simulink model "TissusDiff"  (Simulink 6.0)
settings: Solver=ode45  StartTime=0.0  StopTime=15  RelTol=1e-3
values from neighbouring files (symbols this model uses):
  b = S/Sm    (= 0.1)    [Constantes.m]    (also in ConstantesBck.m)
  C = 1    [Constantes.m]    (also in ConstantesBck.m)
  gk = 36    [Constantes.m]    (also in ConstantesBck.m; sim_hh.m)
  gl = 0.3    [Constantes.m]    (also in ConstantesBck.m; sim_hh.m)
  gna = 120    [Constantes.m]    (also in ConstantesBck.m; sim_hh.m)
  h0 = 0.5961    [Constantes.m]    (also in ConstantesBck.m)
  Istim = 200E-6    (= 0.0002)    [Constantes.m]    (also in ConstantesBck.m = 5e-05)
  m0 = 0.0529    [Constantes.m]    (also in ConstantesBck.m)
  mK = 0    [Constantes.m]    (also in ConstantesBck.m)
  mL = 0    [Constantes.m]    (also in ConstantesBck.m)
  mNa = 0    [Constantes.m]    (also in ConstantesBck.m)
  n0 = 0.3177    [Constantes.m]    (also in ConstantesBck.m)
  rapportIE = 10    [Constantes.m]
  Rext = 2.9E3    (= 2900)    [Constantes.m]    (also in ConstantesBck.m)
  Rint = 2.9E2    (= 290)    [Constantes.m]    (also in ConstantesBck.m = 400)
  Sm = 3.14e-2    (= 0.0314)    [Constantes.m]    (also in ConstantesBck.m = 0.000314)
  Vk = -82    [Constantes.m]    (also in ConstantesBck.m)
  Vl = -59    [Constantes.m]    (also in ConstantesBck.m)
  Vna = 45    [Constantes.m]    (also in ConstantesBck.m)
  Vr = -70    [Constantes.m]    (also in ConstantesBck.m)
undefined symbols (not defined in the file or in its folder): ln

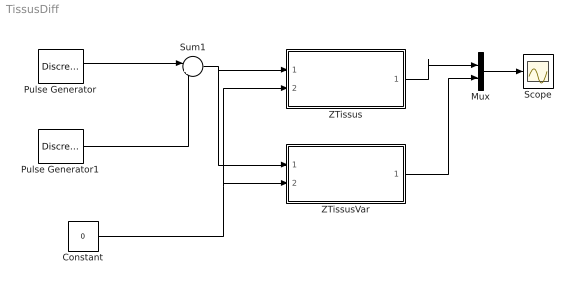
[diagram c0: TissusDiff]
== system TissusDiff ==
  Constant : Constant  Value=0
  Mux : Mux  Inputs=2
  Pulse Generator : DiscretePulseGenerator  PulseType=Time based  Amplitude=-Istim  Period=100  PulseWidth=2  PhaseDelay=2
  Pulse Generator1 : DiscretePulseGenerator  PulseType=Time based  Amplitude=Istim  Period=100  PulseWidth=2  PhaseDelay=4
  Scope : Scope
  Sum1 : Sum  Inputs=|++
  ZTissus : Subsystem
  ZTissusVar : Subsystem
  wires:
  Pulse Generator/1 -> Sum1/1
  Pulse Generator1/1 -> Sum1/2
  Constant/1 -> ZTissus/2(Vref), ZTissusVar/2(Vref)
  Mux/1 -> Scope/1
  Sum1/1 -> ZTissusVar/1(IStim), ZTissus/1(IStim)
  ZTissusVar/1(Vout) -> Mux/2
  ZTissus/1(Vout) -> Mux/1

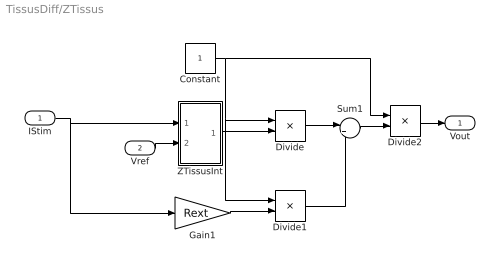
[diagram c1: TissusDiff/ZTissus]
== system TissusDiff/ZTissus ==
  IStim : Inport  Port=1  LatchInput=off
  Vref : Inport  Port=2  LatchInput=off
  Constant : Constant
  Divide : Product  Inputs=*/  OutScaling=2^-10
  Divide1 : Product  Inputs=*/  OutScaling=2^-10
  Divide2 : Product  Inputs=*/  OutScaling=2^-10
  Gain1 : Gain  Gain=Rext
  Sum1 : Sum  Inputs=|++
  ZTissusInt : Subsystem
  Vout : Outport
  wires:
  IStim/1 -> ZTissusInt/1(InStim), Gain1/1
  Constant/1 -> Divide/1, Divide1/1, Divide2/1
  ZTissusInt/1(Vout) -> Divide/2
  Gain1/1 -> Divide1/2
  Divide/1 -> Sum1/1
  Divide1/1 -> Sum1/2
  Sum1/1 -> Divide2/2
  Divide2/1 -> Vout/1
  Vref/1 -> ZTissusInt/2(VRefIn)

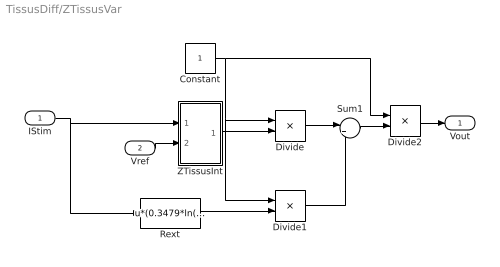
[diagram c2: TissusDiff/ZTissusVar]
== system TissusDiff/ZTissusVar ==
  IStim : Inport  Port=1  LatchInput=off
  Vref : Inport  Port=2  LatchInput=off
  Constant : Constant
  Divide : Product  Inputs=*/  OutScaling=2^-10
  Divide1 : Product  Inputs=*/  OutScaling=2^-10
  Divide2 : Product  Inputs=*/  OutScaling=2^-10
  Rext : Fcn  Expr=u*(0.3479*ln(abs(u)*1E6)+1.3815)*1E3
  Sum1 : Sum  Inputs=|++
  ZTissusInt : Subsystem
  Vout : Outport
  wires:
  IStim/1 -> ZTissusInt/1(InStim), Rext/1
  Constant/1 -> Divide/1, Divide1/1, Divide2/1
  ZTissusInt/1(Vout) -> Divide/2
  Rext/1 -> Divide1/2
  Divide/1 -> Sum1/1
  Divide1/1 -> Sum1/2
  Sum1/1 -> Divide2/2
  Divide2/1 -> Vout/1
  Vref/1 -> ZTissusInt/2(VRefIn)

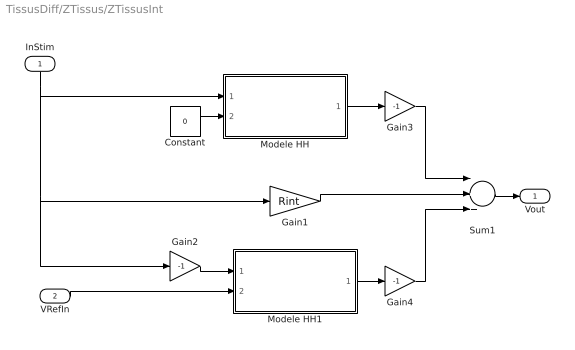
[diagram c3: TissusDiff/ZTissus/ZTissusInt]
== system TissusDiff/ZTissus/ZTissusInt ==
  InStim : Inport  Orientation=down  Port=1  LatchInput=off
  VRefIn : Inport  Port=2  LatchInput=off
  Constant : Constant  Value=0
  Gain1 : Gain  Gain=Rint
  Gain2 : Gain  Gain=-1
  Gain3 : Gain  Gain=-1
  Gain4 : Gain  Gain=-1
  Modele HH : Subsystem
  Modele HH1 : Subsystem
  Sum1 : Sum  Inputs=|+++
  Vout : Outport
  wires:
  Modele HH/1(HHout) -> Gain3/1
  Modele HH1/1(HHout) -> Gain4/1
  Gain1/1 -> Sum1/2
  Gain2/1 -> Modele HH1/1(HHin)
  InStim/1 -> Gain1/1, Gain2/1, Modele HH/1(HHin)
  Constant/1 -> Modele HH/2(VRefIn)
  Sum1/1 -> Vout/1
  VRefIn/1 -> Modele HH1/2(VRefIn)
  Gain3/1 -> Sum1/1
  Gain4/1 -> Sum1/3

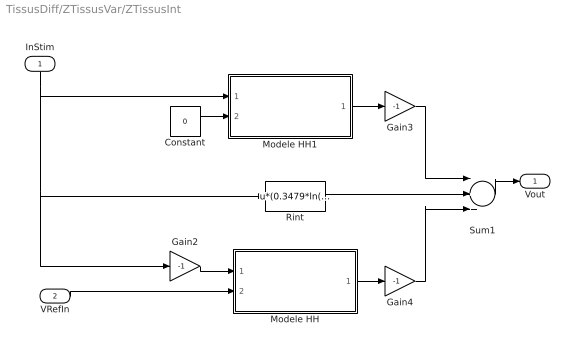
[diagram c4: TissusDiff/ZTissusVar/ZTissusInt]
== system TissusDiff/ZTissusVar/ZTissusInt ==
  InStim : Inport  Orientation=down  Port=1  LatchInput=off
  VRefIn : Inport  Port=2  LatchInput=off
  Constant : Constant  Value=0
  Gain2 : Gain  Gain=-1
  Gain3 : Gain  Gain=-1
  Gain4 : Gain  Gain=-1
  Modele HH : Subsystem
  Modele HH1 : Subsystem
  Rint : Fcn  Expr=u*(0.3479*ln(abs(u)*1E6)+1.3815)*1E3/rapportIE
  Sum1 : Sum  Inputs=|+++
  Vout : Outport
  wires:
  Modele HH1/1(HHout) -> Gain3/1
  Modele HH/1(HHout) -> Gain4/1
  Rint/1 -> Sum1/2
  Gain2/1 -> Modele HH/1(HHin)
  InStim/1 -> Gain2/1, Rint/1, Modele HH1/1(HHin)
  Constant/1 -> Modele HH1/2(VRefIn)
  Sum1/1 -> Vout/1
  VRefIn/1 -> Modele HH/2(VRefIn)
  Gain3/1 -> Sum1/1
  Gain4/1 -> Sum1/3

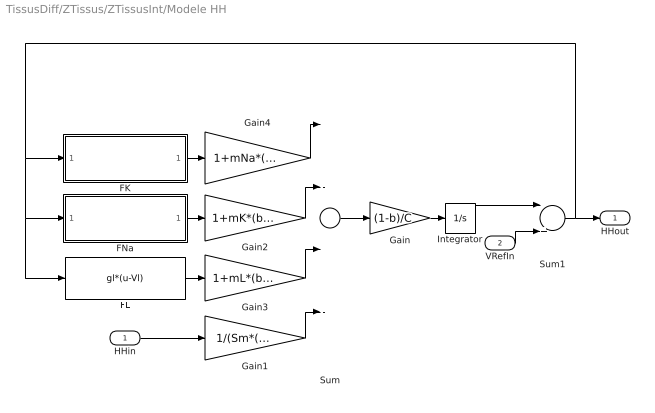
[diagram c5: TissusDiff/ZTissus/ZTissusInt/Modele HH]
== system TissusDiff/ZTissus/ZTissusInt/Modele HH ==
  HHin : Inport  Port=1  LatchInput=off
  VRefIn : Inport  Port=2  LatchInput=off
  FK : Subsystem
  FL : Fcn  Expr=gl*(u-Vl)
  FNa : Subsystem
  Gain : Gain  Gain=(1-b)/C
  Gain1 : Gain  Gain=1/(Sm*(1-b))
  Gain2 : Gain  Gain=1+mK*(b/(1-b))
  Gain3 : Gain  Gain=1+mL*(b/(1-b))
  Gain4 : Gain  Gain=1+mNa*(b/(1-b))
  Integrator : Integrator  InitialCondition=Vr
  Sum : Sum  Inputs=|---+
  Sum1 : Sum  Inputs=|++
  HHout : Outport
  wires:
  Sum/1 -> Gain/1
  Gain/1 -> Integrator/1
  FK/1(FKout) -> Gain4/1
  FNa/1(FNaOut) -> Gain2/1
  FL/1 -> Gain3/1
  HHin/1 -> Gain1/1
  Integrator/1 -> Sum1/1
  Sum1/1 -> HHout/1, FNa/1(FNaIn), FL/1, FK/1(FKIn)
  VRefIn/1 -> Sum1/2
  Gain1/1 -> Sum/4
  Gain4/1 -> Sum/1
  Gain2/1 -> Sum/2
  Gain3/1 -> Sum/3

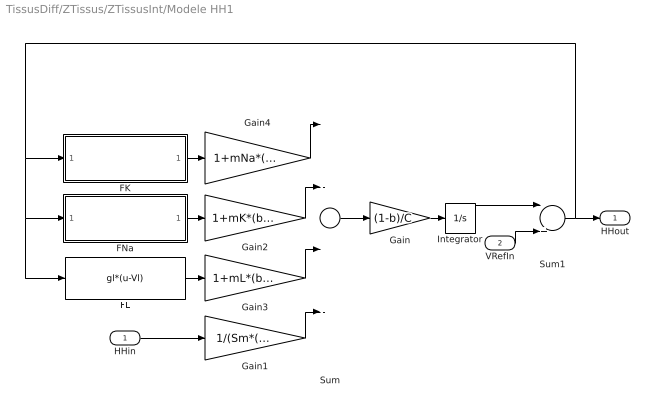
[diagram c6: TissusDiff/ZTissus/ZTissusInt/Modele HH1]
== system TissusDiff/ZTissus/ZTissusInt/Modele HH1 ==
  HHin : Inport  Port=1  LatchInput=off
  VRefIn : Inport  Port=2  LatchInput=off
  FK : Subsystem
  FL : Fcn  Expr=gl*(u-Vl)
  FNa : Subsystem
  Gain : Gain  Gain=(1-b)/C
  Gain1 : Gain  Gain=1/(Sm*(1-b))
  Gain2 : Gain  Gain=1+mK*(b/(1-b))
  Gain3 : Gain  Gain=1+mL*(b/(1-b))
  Gain4 : Gain  Gain=1+mNa*(b/(1-b))
  Integrator : Integrator  InitialCondition=Vr
  Sum : Sum  Inputs=|---+
  Sum1 : Sum  Inputs=|++
  HHout : Outport
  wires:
  Sum/1 -> Gain/1
  Gain/1 -> Integrator/1
  FK/1(FKout) -> Gain4/1
  FNa/1(FNaOut) -> Gain2/1
  FL/1 -> Gain3/1
  HHin/1 -> Gain1/1
  Integrator/1 -> Sum1/1
  Sum1/1 -> HHout/1, FNa/1(FNaIn), FL/1, FK/1(FKIn)
  VRefIn/1 -> Sum1/2
  Gain1/1 -> Sum/4
  Gain4/1 -> Sum/1
  Gain2/1 -> Sum/2
  Gain3/1 -> Sum/3

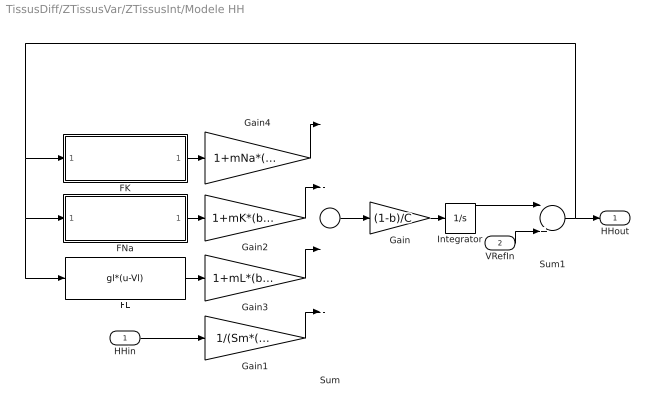
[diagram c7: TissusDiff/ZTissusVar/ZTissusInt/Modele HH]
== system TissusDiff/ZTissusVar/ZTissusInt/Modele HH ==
  HHin : Inport  Port=1  LatchInput=off
  VRefIn : Inport  Port=2  LatchInput=off
  FK : Subsystem
  FL : Fcn  Expr=gl*(u-Vl)
  FNa : Subsystem
  Gain : Gain  Gain=(1-b)/C
  Gain1 : Gain  Gain=1/(Sm*(1-b))
  Gain2 : Gain  Gain=1+mK*(b/(1-b))
  Gain3 : Gain  Gain=1+mL*(b/(1-b))
  Gain4 : Gain  Gain=1+mNa*(b/(1-b))
  Integrator : Integrator  InitialCondition=Vr
  Sum : Sum  Inputs=|---+
  Sum1 : Sum  Inputs=|++
  HHout : Outport
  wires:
  Sum/1 -> Gain/1
  Gain/1 -> Integrator/1
  FK/1(FKout) -> Gain4/1
  FNa/1(FNaOut) -> Gain2/1
  FL/1 -> Gain3/1
  HHin/1 -> Gain1/1
  Integrator/1 -> Sum1/1
  Sum1/1 -> HHout/1, FNa/1(FNaIn), FL/1, FK/1(FKIn)
  VRefIn/1 -> Sum1/2
  Gain1/1 -> Sum/4
  Gain4/1 -> Sum/1
  Gain2/1 -> Sum/2
  Gain3/1 -> Sum/3

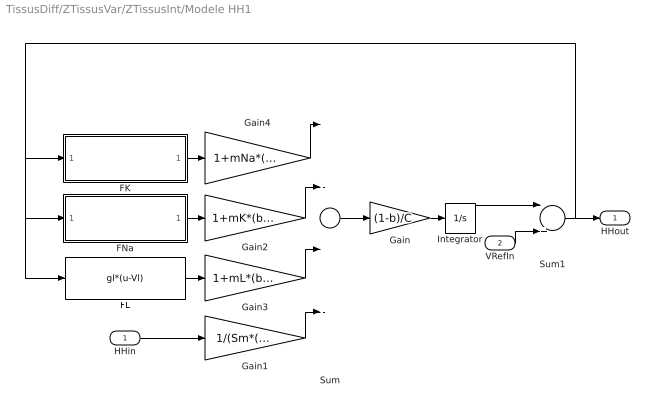
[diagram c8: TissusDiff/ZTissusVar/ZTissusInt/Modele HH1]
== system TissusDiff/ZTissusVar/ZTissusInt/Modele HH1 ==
  HHin : Inport  Port=1  LatchInput=off
  VRefIn : Inport  Port=2  LatchInput=off
  FK : Subsystem
  FL : Fcn  Expr=gl*(u-Vl)
  FNa : Subsystem
  Gain : Gain  Gain=(1-b)/C
  Gain1 : Gain  Gain=1/(Sm*(1-b))
  Gain2 : Gain  Gain=1+mK*(b/(1-b))
  Gain3 : Gain  Gain=1+mL*(b/(1-b))
  Gain4 : Gain  Gain=1+mNa*(b/(1-b))
  Integrator : Integrator  InitialCondition=Vr
  Sum : Sum  Inputs=|---+
  Sum1 : Sum  Inputs=|++
  HHout : Outport
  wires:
  Sum/1 -> Gain/1
  Gain/1 -> Integrator/1
  FK/1(FKout) -> Gain4/1
  FNa/1(FNaOut) -> Gain2/1
  FL/1 -> Gain3/1
  HHin/1 -> Gain1/1
  Integrator/1 -> Sum1/1
  Sum1/1 -> HHout/1, FNa/1(FNaIn), FL/1, FK/1(FKIn)
  VRefIn/1 -> Sum1/2
  Gain1/1 -> Sum/4
  Gain4/1 -> Sum/1
  Gain2/1 -> Sum/2
  Gain3/1 -> Sum/3

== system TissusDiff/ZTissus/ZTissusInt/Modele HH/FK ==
  note: gkm
  note: (Vm-Vk0)
  FKIn : Inport  Port=1  LatchInput=off
  (Vm-Vk0) : Fcn  Expr=(u-Vk)
  Product : Product
  n(Vm) : Subsystem
  n^4 : Fcn  Expr=gk*(u^4)
  FKout : Outport  InitialOutput=0
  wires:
  n(Vm)/1(n) -> n^4/1
  (Vm-Vk0)/1 -> Product/2
  Product/1 -> FKout/1
  n^4/1 -> Product/1
  FKIn/1 -> n(Vm)/1(Vm), (Vm-Vk0)/1

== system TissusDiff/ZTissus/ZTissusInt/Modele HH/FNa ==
  note: gNa*m^3
  note: m
  note: h
  note: gNam
  note: (Vm-VNa0)
  FNaIn : Inport  Port=1  LatchInput=off
  (Vm-VNa0) : Fcn  Expr=(u-Vna)
  Product : Product
  Product1 : Product
  gna*m^3 : Fcn  Expr=gna*u^3
  h(Vm) : Subsystem
  m(Vm) : Subsystem
  FNaOut : Outport  InitialOutput=0
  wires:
  (Vm-VNa0)/1 -> Product1/2
  gna*m^3/1 -> Product/1
  Product1/1 -> FNaOut/1
  FNaIn/1 -> m(Vm)/1(Vm), h(Vm)/1(Vm), (Vm-VNa0)/1
  m(Vm)/1(n) -> gna*m^3/1
  h(Vm)/1(h) -> Product/2
  Product/1 -> Product1/1

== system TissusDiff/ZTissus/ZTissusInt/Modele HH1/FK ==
  note: gkm
  note: (Vm-Vk0)
  FKIn : Inport  Port=1  LatchInput=off
  (Vm-Vk0) : Fcn  Expr=(u-Vk)
  Product : Product
  n(Vm) : Subsystem
  n^4 : Fcn  Expr=gk*(u^4)
  FKout : Outport  InitialOutput=0
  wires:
  n(Vm)/1(n) -> n^4/1
  (Vm-Vk0)/1 -> Product/2
  Product/1 -> FKout/1
  n^4/1 -> Product/1
  FKIn/1 -> n(Vm)/1(Vm), (Vm-Vk0)/1

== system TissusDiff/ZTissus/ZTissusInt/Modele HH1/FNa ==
  note: gNa*m^3
  note: m
  note: h
  note: gNam
  note: (Vm-VNa0)
  FNaIn : Inport  Port=1  LatchInput=off
  (Vm-VNa0) : Fcn  Expr=(u-Vna)
  Product : Product
  Product1 : Product
  gna*m^3 : Fcn  Expr=gna*u^3
  h(Vm) : Subsystem
  m(Vm) : Subsystem
  FNaOut : Outport  InitialOutput=0
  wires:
  (Vm-VNa0)/1 -> Product1/2
  gna*m^3/1 -> Product/1
  Product1/1 -> FNaOut/1
  FNaIn/1 -> m(Vm)/1(Vm), h(Vm)/1(Vm), (Vm-VNa0)/1
  m(Vm)/1(n) -> gna*m^3/1
  h(Vm)/1(h) -> Product/2
  Product/1 -> Product1/1

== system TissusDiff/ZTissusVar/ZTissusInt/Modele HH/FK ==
  note: gkm
  note: (Vm-Vk0)
  FKIn : Inport  Port=1  LatchInput=off
  (Vm-Vk0) : Fcn  Expr=(u-Vk)
  Product : Product
  n(Vm) : Subsystem
  n^4 : Fcn  Expr=gk*(u^4)
  FKout : Outport  InitialOutput=0
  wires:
  n(Vm)/1(n) -> n^4/1
  (Vm-Vk0)/1 -> Product/2
  Product/1 -> FKout/1
  n^4/1 -> Product/1
  FKIn/1 -> n(Vm)/1(Vm), (Vm-Vk0)/1

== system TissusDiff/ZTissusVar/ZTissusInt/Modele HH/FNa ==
  note: gNa*m^3
  note: m
  note: h
  note: gNam
  note: (Vm-VNa0)
  FNaIn : Inport  Port=1  LatchInput=off
  (Vm-VNa0) : Fcn  Expr=(u-Vna)
  Product : Product
  Product1 : Product
  gna*m^3 : Fcn  Expr=gna*u^3
  h(Vm) : Subsystem
  m(Vm) : Subsystem
  FNaOut : Outport  InitialOutput=0
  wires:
  (Vm-VNa0)/1 -> Product1/2
  gna*m^3/1 -> Product/1
  Product1/1 -> FNaOut/1
  FNaIn/1 -> m(Vm)/1(Vm), h(Vm)/1(Vm), (Vm-VNa0)/1
  m(Vm)/1(n) -> gna*m^3/1
  h(Vm)/1(h) -> Product/2
  Product/1 -> Product1/1

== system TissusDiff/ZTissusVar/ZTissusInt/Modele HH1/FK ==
  note: gkm
  note: (Vm-Vk0)
  FKIn : Inport  Port=1  LatchInput=off
  (Vm-Vk0) : Fcn  Expr=(u-Vk)
  Product : Product
  n(Vm) : Subsystem
  n^4 : Fcn  Expr=gk*(u^4)
  FKout : Outport  InitialOutput=0
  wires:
  n(Vm)/1(n) -> n^4/1
  (Vm-Vk0)/1 -> Product/2
  Product/1 -> FKout/1
  n^4/1 -> Product/1
  FKIn/1 -> n(Vm)/1(Vm), (Vm-Vk0)/1

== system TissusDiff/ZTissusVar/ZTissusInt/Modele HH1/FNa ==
  note: gNa*m^3
  note: m
  note: h
  note: gNam
  note: (Vm-VNa0)
  FNaIn : Inport  Port=1  LatchInput=off
  (Vm-VNa0) : Fcn  Expr=(u-Vna)
  Product : Product
  Product1 : Product
  gna*m^3 : Fcn  Expr=gna*u^3
  h(Vm) : Subsystem
  m(Vm) : Subsystem
  FNaOut : Outport  InitialOutput=0
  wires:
  (Vm-VNa0)/1 -> Product1/2
  gna*m^3/1 -> Product/1
  Product1/1 -> FNaOut/1
  FNaIn/1 -> m(Vm)/1(Vm), h(Vm)/1(Vm), (Vm-VNa0)/1
  m(Vm)/1(n) -> gna*m^3/1
  h(Vm)/1(h) -> Product/2
  Product/1 -> Product1/1

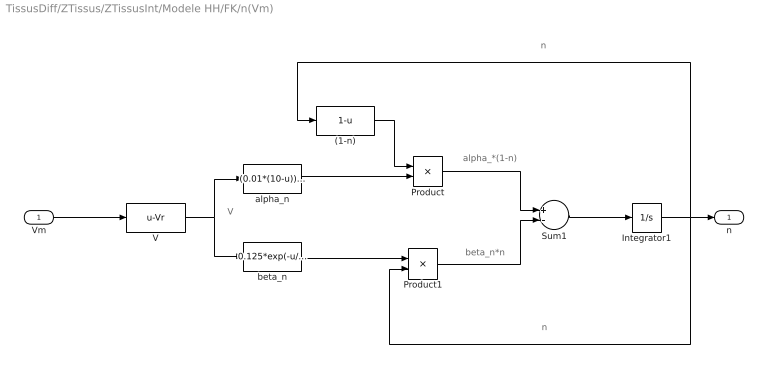
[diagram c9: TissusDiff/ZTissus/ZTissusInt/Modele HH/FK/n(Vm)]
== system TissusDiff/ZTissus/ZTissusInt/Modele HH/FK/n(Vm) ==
  note: V
  note: alpha_*(1-n)
  note: beta_n*n
  note: n
  note: n
  Vm : Inport  Port=1  LatchInput=off
  (1-n) : Fcn  Expr=1-u
  Integrator1 : Integrator  InitialCondition=n0
  Product : Product
  Product1 : Product
  Sum1 : Sum  Inputs=+-
  V : Fcn  Expr=u-Vr
  alpha_n : Fcn  Expr=(0.01*(10-u))/(exp((10-u)/10)-1)
  beta_n : Fcn  Expr=0.125*exp(-u/80)
  n : Outport  InitialOutput=0
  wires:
  V/1 -> alpha_n/1, beta_n/1
  alpha_n/1 -> Product/2
  (1-n)/1 -> Product/1
  beta_n/1 -> Product1/1
  Product/1 -> Sum1/1
  Product1/1 -> Sum1/2
  Sum1/1 -> Integrator1/1
  Integrator1/1 -> (1-n)/1, Product1/2, n/1
  Vm/1 -> V/1

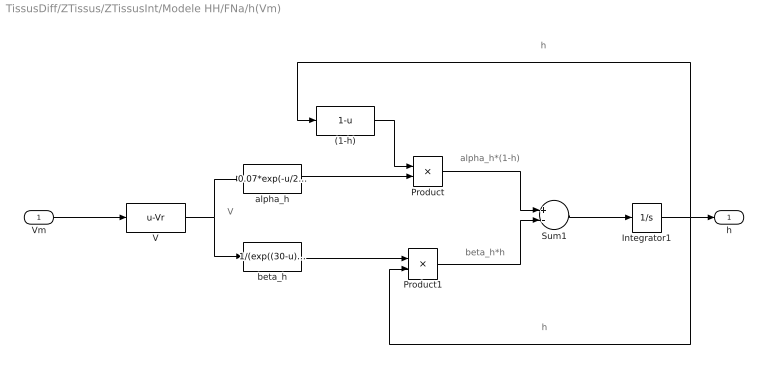
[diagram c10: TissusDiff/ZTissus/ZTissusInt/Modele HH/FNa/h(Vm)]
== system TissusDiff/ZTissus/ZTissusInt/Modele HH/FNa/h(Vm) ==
  note: h
  note: h
  note: beta_h*h
  note: alpha_h*(1-h)
  note: V
  Vm : Inport  Port=1  LatchInput=off
  (1-h) : Fcn  Expr=1-u
  Integrator1 : Integrator  InitialCondition=h0
  Product : Product
  Product1 : Product
  Sum1 : Sum  Inputs=+-
  V : Fcn  Expr=u-Vr
  alpha_h : Fcn  Expr=0.07*exp(-u/20)
  beta_h : Fcn  Expr=1/(exp((30-u)/10)+1)
  h : Outport  InitialOutput=0
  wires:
  Vm/1 -> V/1
  Integrator1/1 -> h/1, Product1/2, (1-h)/1
  Sum1/1 -> Integrator1/1
  Product1/1 -> Sum1/2
  Product/1 -> Sum1/1
  beta_h/1 -> Product1/1
  (1-h)/1 -> Product/1
  alpha_h/1 -> Product/2
  V/1 -> beta_h/1, alpha_h/1

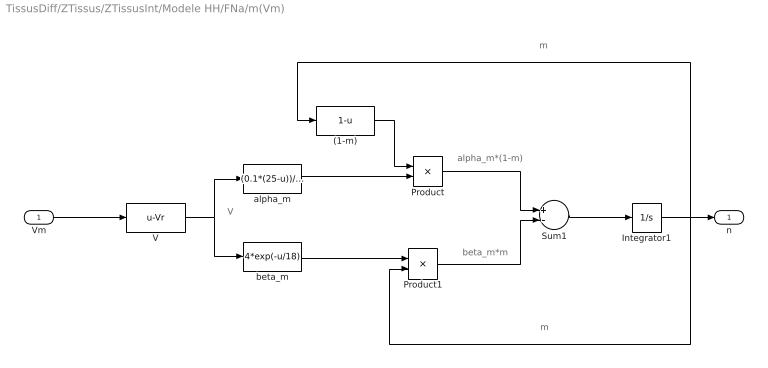
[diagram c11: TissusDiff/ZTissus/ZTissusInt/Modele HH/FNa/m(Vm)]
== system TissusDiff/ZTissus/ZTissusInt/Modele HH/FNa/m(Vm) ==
  note: m
  note: m
  note: beta_m*m
  note: alpha_m*(1-m)
  note: V
  Vm : Inport  Port=1  LatchInput=off
  (1-m) : Fcn  Expr=1-u
  Integrator1 : Integrator  InitialCondition=m0
  Product : Product
  Product1 : Product
  Sum1 : Sum  Inputs=+-
  V : Fcn  Expr=u-Vr
  alpha_m : Fcn  Expr=(0.1*(25-u))/(exp((25-u)/10)-1)
  beta_m : Fcn  Expr=4*exp(-u/18)
  n : Outport  InitialOutput=0
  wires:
  Vm/1 -> V/1
  Integrator1/1 -> n/1, Product1/2, (1-m)/1
  Sum1/1 -> Integrator1/1
  Product1/1 -> Sum1/2
  Product/1 -> Sum1/1
  beta_m/1 -> Product1/1
  (1-m)/1 -> Product/1
  alpha_m/1 -> Product/2
  V/1 -> beta_m/1, alpha_m/1

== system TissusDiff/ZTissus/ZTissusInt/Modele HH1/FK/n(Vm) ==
  note: V
  note: alpha_*(1-n)
  note: beta_n*n
  note: n
  note: n
  Vm : Inport  Port=1  LatchInput=off
  (1-n) : Fcn  Expr=1-u
  Integrator1 : Integrator  InitialCondition=n0
  Product : Product
  Product1 : Product
  Sum1 : Sum  Inputs=+-
  V : Fcn  Expr=u-Vr
  alpha_n : Fcn  Expr=(0.01*(10-u))/(exp((10-u)/10)-1)
  beta_n : Fcn  Expr=0.125*exp(-u/80)
  n : Outport  InitialOutput=0
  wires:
  V/1 -> alpha_n/1, beta_n/1
  alpha_n/1 -> Product/2
  (1-n)/1 -> Product/1
  beta_n/1 -> Product1/1
  Product/1 -> Sum1/1
  Product1/1 -> Sum1/2
  Sum1/1 -> Integrator1/1
  Integrator1/1 -> (1-n)/1, Product1/2, n/1
  Vm/1 -> V/1

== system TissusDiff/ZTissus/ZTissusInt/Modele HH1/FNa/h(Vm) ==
  note: h
  note: h
  note: beta_h*h
  note: alpha_h*(1-h)
  note: V
  Vm : Inport  Port=1  LatchInput=off
  (1-h) : Fcn  Expr=1-u
  Integrator1 : Integrator  InitialCondition=h0
  Product : Product
  Product1 : Product
  Sum1 : Sum  Inputs=+-
  V : Fcn  Expr=u-Vr
  alpha_h : Fcn  Expr=0.07*exp(-u/20)
  beta_h : Fcn  Expr=1/(exp((30-u)/10)+1)
  h : Outport  InitialOutput=0
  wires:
  Vm/1 -> V/1
  Integrator1/1 -> h/1, Product1/2, (1-h)/1
  Sum1/1 -> Integrator1/1
  Product1/1 -> Sum1/2
  Product/1 -> Sum1/1
  beta_h/1 -> Product1/1
  (1-h)/1 -> Product/1
  alpha_h/1 -> Product/2
  V/1 -> beta_h/1, alpha_h/1

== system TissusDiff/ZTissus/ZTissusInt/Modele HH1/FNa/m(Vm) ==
  note: m
  note: m
  note: beta_m*m
  note: alpha_m*(1-m)
  note: V
  Vm : Inport  Port=1  LatchInput=off
  (1-m) : Fcn  Expr=1-u
  Integrator1 : Integrator  InitialCondition=m0
  Product : Product
  Product1 : Product
  Sum1 : Sum  Inputs=+-
  V : Fcn  Expr=u-Vr
  alpha_m : Fcn  Expr=(0.1*(25-u))/(exp((25-u)/10)-1)
  beta_m : Fcn  Expr=4*exp(-u/18)
  n : Outport  InitialOutput=0
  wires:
  Vm/1 -> V/1
  Integrator1/1 -> n/1, Product1/2, (1-m)/1
  Sum1/1 -> Integrator1/1
  Product1/1 -> Sum1/2
  Product/1 -> Sum1/1
  beta_m/1 -> Product1/1
  (1-m)/1 -> Product/1
  alpha_m/1 -> Product/2
  V/1 -> beta_m/1, alpha_m/1

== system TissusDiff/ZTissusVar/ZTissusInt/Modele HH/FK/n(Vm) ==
  note: V
  note: alpha_*(1-n)
  note: beta_n*n
  note: n
  note: n
  Vm : Inport  Port=1  LatchInput=off
  (1-n) : Fcn  Expr=1-u
  Integrator1 : Integrator  InitialCondition=n0
  Product : Product
  Product1 : Product
  Sum1 : Sum  Inputs=+-
  V : Fcn  Expr=u-Vr
  alpha_n : Fcn  Expr=(0.01*(10-u))/(exp((10-u)/10)-1)
  beta_n : Fcn  Expr=0.125*exp(-u/80)
  n : Outport  InitialOutput=0
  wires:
  V/1 -> alpha_n/1, beta_n/1
  alpha_n/1 -> Product/2
  (1-n)/1 -> Product/1
  beta_n/1 -> Product1/1
  Product/1 -> Sum1/1
  Product1/1 -> Sum1/2
  Sum1/1 -> Integrator1/1
  Integrator1/1 -> (1-n)/1, Product1/2, n/1
  Vm/1 -> V/1

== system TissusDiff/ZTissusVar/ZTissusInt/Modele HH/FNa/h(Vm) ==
  note: h
  note: h
  note: beta_h*h
  note: alpha_h*(1-h)
  note: V
  Vm : Inport  Port=1  LatchInput=off
  (1-h) : Fcn  Expr=1-u
  Integrator1 : Integrator  InitialCondition=h0
  Product : Product
  Product1 : Product
  Sum1 : Sum  Inputs=+-
  V : Fcn  Expr=u-Vr
  alpha_h : Fcn  Expr=0.07*exp(-u/20)
  beta_h : Fcn  Expr=1/(exp((30-u)/10)+1)
  h : Outport  InitialOutput=0
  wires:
  Vm/1 -> V/1
  Integrator1/1 -> h/1, Product1/2, (1-h)/1
  Sum1/1 -> Integrator1/1
  Product1/1 -> Sum1/2
  Product/1 -> Sum1/1
  beta_h/1 -> Product1/1
  (1-h)/1 -> Product/1
  alpha_h/1 -> Product/2
  V/1 -> beta_h/1, alpha_h/1

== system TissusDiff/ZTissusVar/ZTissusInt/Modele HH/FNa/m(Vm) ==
  note: m
  note: m
  note: beta_m*m
  note: alpha_m*(1-m)
  note: V
  Vm : Inport  Port=1  LatchInput=off
  (1-m) : Fcn  Expr=1-u
  Integrator1 : Integrator  InitialCondition=m0
  Product : Product
  Product1 : Product
  Sum1 : Sum  Inputs=+-
  V : Fcn  Expr=u-Vr
  alpha_m : Fcn  Expr=(0.1*(25-u))/(exp((25-u)/10)-1)
  beta_m : Fcn  Expr=4*exp(-u/18)
  n : Outport  InitialOutput=0
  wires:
  Vm/1 -> V/1
  Integrator1/1 -> n/1, Product1/2, (1-m)/1
  Sum1/1 -> Integrator1/1
  Product1/1 -> Sum1/2
  Product/1 -> Sum1/1
  beta_m/1 -> Product1/1
  (1-m)/1 -> Product/1
  alpha_m/1 -> Product/2
  V/1 -> beta_m/1, alpha_m/1

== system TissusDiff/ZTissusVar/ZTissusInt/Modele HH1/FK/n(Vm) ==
  note: V
  note: alpha_*(1-n)
  note: beta_n*n
  note: n
  note: n
  Vm : Inport  Port=1  LatchInput=off
  (1-n) : Fcn  Expr=1-u
  Integrator1 : Integrator  InitialCondition=n0
  Product : Product
  Product1 : Product
  Sum1 : Sum  Inputs=+-
  V : Fcn  Expr=u-Vr
  alpha_n : Fcn  Expr=(0.01*(10-u))/(exp((10-u)/10)-1)
  beta_n : Fcn  Expr=0.125*exp(-u/80)
  n : Outport  InitialOutput=0
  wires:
  V/1 -> alpha_n/1, beta_n/1
  alpha_n/1 -> Product/2
  (1-n)/1 -> Product/1
  beta_n/1 -> Product1/1
  Product/1 -> Sum1/1
  Product1/1 -> Sum1/2
  Sum1/1 -> Integrator1/1
  Integrator1/1 -> (1-n)/1, Product1/2, n/1
  Vm/1 -> V/1

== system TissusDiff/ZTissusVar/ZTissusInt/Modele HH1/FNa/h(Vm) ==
  note: h
  note: h
  note: beta_h*h
  note: alpha_h*(1-h)
  note: V
  Vm : Inport  Port=1  LatchInput=off
  (1-h) : Fcn  Expr=1-u
  Integrator1 : Integrator  InitialCondition=h0
  Product : Product
  Product1 : Product
  Sum1 : Sum  Inputs=+-
  V : Fcn  Expr=u-Vr
  alpha_h : Fcn  Expr=0.07*exp(-u/20)
  beta_h : Fcn  Expr=1/(exp((30-u)/10)+1)
  h : Outport  InitialOutput=0
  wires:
  Vm/1 -> V/1
  Integrator1/1 -> h/1, Product1/2, (1-h)/1
  Sum1/1 -> Integrator1/1
  Product1/1 -> Sum1/2
  Product/1 -> Sum1/1
  beta_h/1 -> Product1/1
  (1-h)/1 -> Product/1
  alpha_h/1 -> Product/2
  V/1 -> beta_h/1, alpha_h/1

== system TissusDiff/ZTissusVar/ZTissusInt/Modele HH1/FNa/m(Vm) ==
  note: m
  note: m
  note: beta_m*m
  note: alpha_m*(1-m)
  note: V
  Vm : Inport  Port=1  LatchInput=off
  (1-m) : Fcn  Expr=1-u
  Integrator1 : Integrator  InitialCondition=m0
  Product : Product
  Product1 : Product
  Sum1 : Sum  Inputs=+-
  V : Fcn  Expr=u-Vr
  alpha_m : Fcn  Expr=(0.1*(25-u))/(exp((25-u)/10)-1)
  beta_m : Fcn  Expr=4*exp(-u/18)
  n : Outport  InitialOutput=0
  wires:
  Vm/1 -> V/1
  Integrator1/1 -> n/1, Product1/2, (1-m)/1
  Sum1/1 -> Integrator1/1
  Product1/1 -> Sum1/2
  Product/1 -> Sum1/1
  beta_m/1 -> Product1/1
  (1-m)/1 -> Product/1
  alpha_m/1 -> Product/2
  V/1 -> beta_m/1, alpha_m/1
